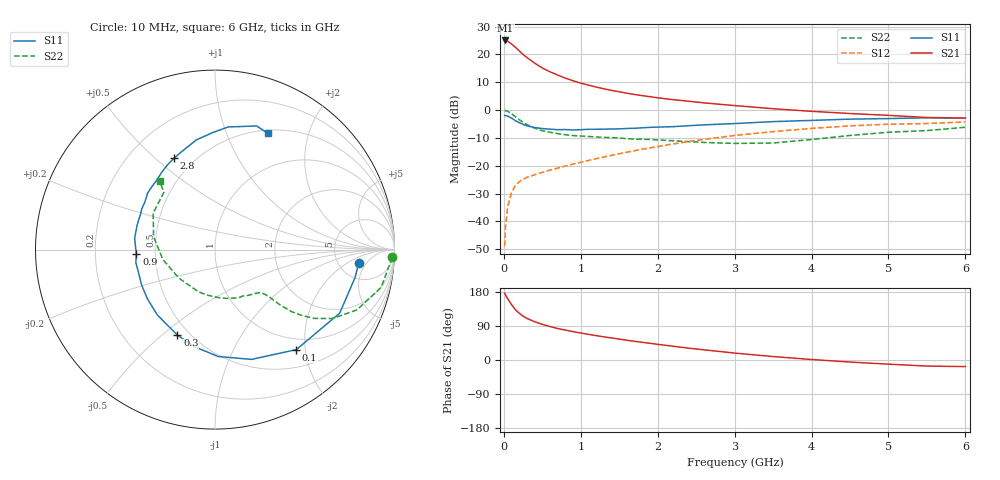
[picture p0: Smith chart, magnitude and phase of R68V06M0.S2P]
! SIEMENS Small Signal Semiconductors
! BFR193
! Si NPN RF Bipolar Junction Transistor in SOT23
! VCE = 8 V  IC = 6 mA
! Common Emitter S-Parameters:  May  1996
# GHz  S  MA  R  50
!  f  S11  S21  S12  S22
! GHz  MAG  ANG  MAG  ANG  MAG  ANG  MAG  ANG
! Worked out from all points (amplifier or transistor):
!   36 points, 10 MHz to 6 GHz, reference 50 ohm
!   highest |S21| = 25.0 dB at 20 MHz (marker M1)
!   |S21| within 3 dB of that: start of sweep to 171.5 MHz
!   unconditionally stable (mu >= 1): 870.3 MHz to 2.031 GHz
!   at 250 MHz: K = 0.47, MSG = 22.4 dB, |S12| = -24.9 dB
!   at 1.4 GHz: K = 1.05, MAG = 10.2 dB, |S12| = -16.3 dB
!   at 6 GHz: K = 0.95, MSG = 0.7 dB, |S12| = -4.3 dB
!   lowest NFmin = 1.20 dB at 450 MHz
!   S11 on the Smith chart (normalised r, x): 10 MHz: 7.76, -3.32; 100 MHz: 0.79, -1.83; 300 MHz: 0.43, -0.56; 900 MHz: 0.39, -0.02; 2.8 GHz: 0.39, +0.58; 6 GHz: 0.54, +1.41
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0.01  0.8039 -5.4  17.63 176.4  0.0036 88.6  0.9876 -2.5
0.02  0.7959 -11.2  17.78 172.2  0.0076 85.8  0.9749 -5.2
0.05  0.7798 -27.0  17.23 161.7  0.0185 76.1  0.9496 -12.8
0.1  0.7181 -50.9  15.37 146.2  0.0333 66.3  0.8592 -23.0
0.15  0.6447 -71.6  13.43 132.8  0.0441 58.8  0.7588 -30.4
0.2  0.5957 -88.3  11.55 123.4  0.0518 54.7  0.6719 -34.8
0.25  0.5534 -101.8  9.967 115.8  0.0571 51.9  0.6036 -37.3
0.3  0.5206 -113.7  8.773 109.7  0.0619 50.8  0.5495 -39.0
0.4  0.4856 -131.4  6.983 101.1  0.0691 50.0  0.4727 -40.4
0.5  0.466 -143.8  5.694 94.1  0.076 50.8  0.4266 -40.8
0.6  0.4539 -154.4  4.863 88.3  0.0836 52.0  0.3991 -41.1
0.7  0.4446 -163.5  4.248 83.1  0.0907 53.6  0.3774 -41.7
0.9  0.4388 -176.9  3.353 74.9  0.1075 56.6  0.3483 -43.3
1.1  0.4518 172.1  2.803 67.7  0.1245 58.2  0.3358 -46.5
1.3  0.4546 162.5  2.407 61.1  0.144 59.1  0.3236 -49.9
1.6  0.4673 150.7  2.006 52.1  0.1751 59.6  0.307 -56.9
2.2  0.5034 130.8  1.539 36.3  0.2463 56.6  0.2812 -75.2
2.8  0.5573 114.2  1.272 22.6  0.3232 50.5  0.2566 -101.4
3.5  0.6202 99.6  1.057 9.1  0.4105 40.2  0.2563 -141.7
4.5  0.6876 83.8  0.867 -5.4  0.52 24.4  0.35 168.0
5.5  0.7271 71.4  0.735 -16.0  0.573 7.6  0.4284 131.6
6  0.7118 65.7  0.719 -17.4  0.6121 2.8  0.491 129.0
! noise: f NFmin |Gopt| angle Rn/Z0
0.45  1.2  0.25  114  0.13
0.9  1.25  0.37  150  0.12
1.8  2  0.55  -158  0.12
